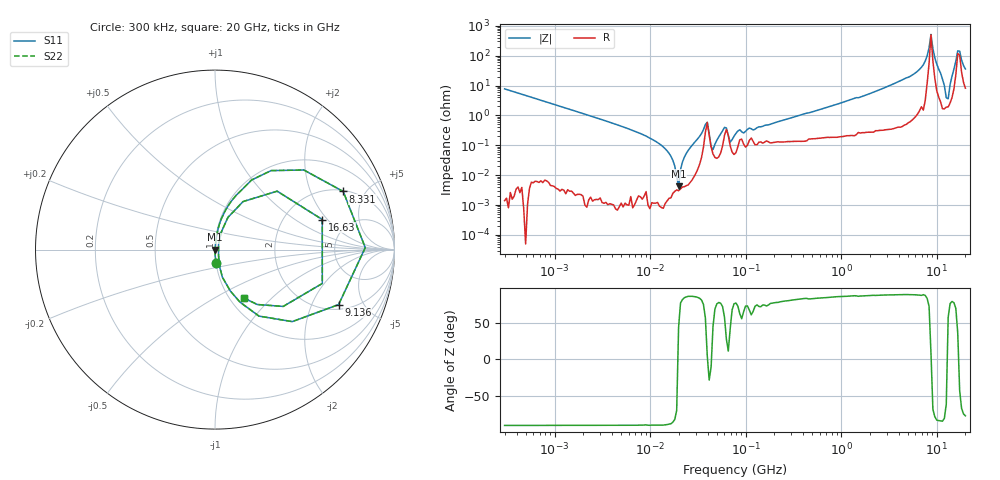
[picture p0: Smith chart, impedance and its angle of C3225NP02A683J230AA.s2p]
! S-parameter Generated by TDK Corporation
! Copyright(C) 2015 TDK Corporation.
! All Rights Reserved.
! TDK P/N: C3225NP02A683J230AA (Multilayer Ceramic Chip Capacitors)
! Property: C=68nF
! Size(LxWxT): 3.2x2.5x2.3mm, 0.126x0.098x0.091inches
! Model Type: s2p (Touchstone File Format Version 1.0)
! Frequency: DC=Yes Start=0.3MHz Stop=20000MHz 243points Log-sweep
! Note:
! Model Generated on Jun. 23, 2015
! Hash(MD5):
! Port Assignments:
!  1 ---| |--- 2
! Applicable Conditions:
!  Temperature = 25 degC
!  DC Bias Voltage = 0 V
!  Small Signal Operation
! Terms and conditions regarding TDK Simulation Models
! (1)This simulation model is being provided solely for informational purposes. Please refer to the specifications of the products in terms of detailed characteristics of such products.
! (2)In no event shall TDK Corporation of any of its subsidiaries be liable for any loss or damage arising, directly or indirectly,
!  From any information contained in this simulation model, including, but not limited to loss or damages arising from any inaccuracies, omissions or errors in connection with such information.
! (3)Any and all copyrights on this simulation model are owned by TDK Corporation.
!  Duplication or redistribution of this simulation model without prior written permission from TDK Corporation is prohibited.
! (4)This simulation model is subject to any modification or change without any prior notice.
! (5)Neither TDK Corporation nor any of its subsidiaries shall make any warranty, express or implied,
!  Including but not limited to the correctness, implied warranties of merchantability and fitness for a particular purpose with respect to this simulation models.
! (6)The use of this simulation model shall be deemed to have consented to the terms and conditions hereof.
# MHz S MA R 50
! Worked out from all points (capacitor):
!   242 points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, 300 kHz to 20 GHz, reference 50 ohm
!   read as one part in series: C = 68.7 nF near 314.2 kHz
!   lowest |Z| = 4.19 mohm at 19.89 MHz (marker M1)
!   series resonance near 19.66 MHz, so ESL is about 950 pH
!   S11 on the Smith chart (normalised r, x): 300 kHz: 1.00, -0.15; 8.331 GHz: 2.06, +3.47; 9.136 GHz: 2.26, -3.21; 16.63 GHz: 3.24, +1.76; 20 GHz: 1.16, -0.70
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0.3  0.07692 -85.6  0.997 4.4  0.997 4.4  0.07692 -85.6
1.985118  0.01151 -89.2  0.9999 0.7  0.9999 0.7  0.01151 -89.2
12.54397  0.001112 -89.5  1 0.1  1 0.1  0.001112 -89.5
19.88828  4.141e-05 44.2  1 -0.0  1 -0.0  4.141e-05 44.2
23.91454  0.0005318 85.2  1 -0.0  1 -0.0  0.0005318 85.2
39.70457  0.005823 4.7  0.9942 -0.0  0.9942 -0.0  0.005823 4.7
45.59205  0.0007245 45.2  0.9995 -0.0  0.9995 -0.0  0.0007245 45.2
60.11549  0.003967 57.5  0.9979 -0.2  0.9979 -0.2  0.003967 57.5
69.02956  0.001278 42.5  0.9991 -0.0  0.9991 -0.0  0.001278 42.5
79.26541  0.002492 76.7  0.9994 -0.1  0.9994 -0.1  0.002492 76.7
500.8786  0.01314 82.0  0.9983 -0.7  0.9983 -0.7  0.01314 82.0
3165.055  0.0962 82.5  0.992 -5.5  0.992 -5.5  0.0962 82.5
6616.689  0.3235 68.8  0.9329 -18.9  0.9329 -18.9  0.3235 68.8
8331.474  0.7843 24.4  0.4285 -48.2  0.4285 -48.2  0.7843 24.4
8724.45  0.8373 0.7  0.1642 -7.7  0.1642 -7.7  0.8373 0.7
9135.962  0.7537 -24.0  0.4329 44.0  0.4329 44.0  0.7537 -24.0
10490.66  0.3237 -64.6  0.909 18.8  0.909 18.8  0.3237 -64.6
13209.43  0.0352 55.7  0.9806 -1.7  0.9806 -1.7  0.0352 55.7
14484.93  0.1933 68.1  0.9447 -10.9  0.9447 -10.9  0.1933 68.1
16632.79  0.6207 15.7  0.4294 -20.5  0.4294 -20.5  0.6207 15.7
18238.85  0.4947 -39.8  0.6939 26.9  0.6939 26.9  0.4947 -39.8
20000  0.3154 -59.0  0.8801 17.9  0.8801 17.9  0.3154 -59.0
